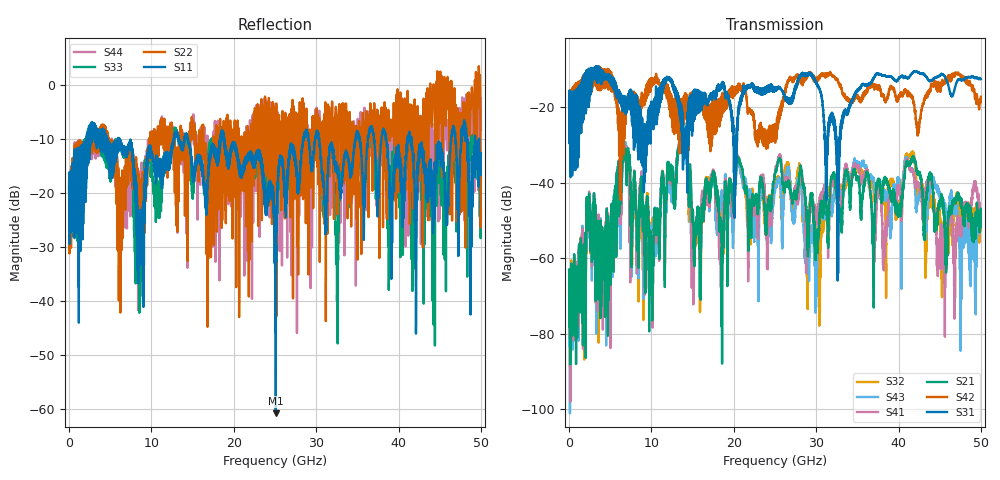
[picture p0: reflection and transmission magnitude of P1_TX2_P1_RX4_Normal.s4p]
!Keysight Technologies,N5225B,MY57041031,A.13.20.10
!Date: Friday, May 31, 2019 11:18:54
!Correction: S11(Full 4 Port(1,2,3,4))
!S12(Full 4 Port(1,2,3,4))
!S13(Full 4 Port(1,2,3,4))
!S14(Full 4 Port(1,2,3,4))
!S21(Full 4 Port(1,2,3,4))
!S22(Full 4 Port(1,2,3,4))
!S23(Full 4 Port(1,2,3,4))
!S24(Full 4 Port(1,2,3,4))
!S31(Full 4 Port(1,2,3,4))
!S32(Full 4 Port(1,2,3,4))
!S33(Full 4 Port(1,2,3,4))
!S34(Full 4 Port(1,2,3,4))
!S41(Full 4 Port(1,2,3,4))
!S42(Full 4 Port(1,2,3,4))
!S43(Full 4 Port(1,2,3,4))
!S44(Full 4 Port(1,2,3,4))
!S4P File: Measurements: <S11,S12,S13,S14>,
!<S21,S22,S23,S24>,
!<S31,S32,S33,S34>,
!<S41,S42,S43,S44>:
# Hz S  dB  R 50.0
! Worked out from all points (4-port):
!   5000 points, 10 MHz to 50 GHz, reference 50 ohm
!   strongest paths, dB at 10 MHz, 12.51 GHz, 25.01 GHz, 37.51 GHz, 50 GHz:
!     S31: -19.5, -13.0, -15.4, -11.1, -12.6
!     S42: -19.3, -19.5, -26.1, -14.9, -17.3
!     S21: -63.0, -38.6, -37.9, -39.2, -47.6
!     S41: -65.3, -39.8, -37.5, -42.3, -48.5
!     S43: -66.8, -44.0, -42.1, -42.7, -48.7
!     S32: -68.5, -42.4, -40.1, -39.7, -50.0
!   lowest |S11| = -60.7 dB at 25.1 GHz (marker M1), VSWR 1.00, Z = 49.9 - j0.0116 ohm
!   |S11| at or under -10 dB: 6.091 GHz to 12.71 GHz (6.616 GHz wide, 70.4 % of centre); 18.82 GHz to 28.43 GHz (9.605 GHz wide, 40.7 % of centre); 41.58 GHz to 46.39 GHz (4.81 GHz wide, 10.9 % of centre)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
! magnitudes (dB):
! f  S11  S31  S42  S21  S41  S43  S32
! 10 MHz  -19.9  -19.5  -19.3  -63.0  -65.3  -66.8  -68.5
! 6.74 GHz  -12.2  -19.2  -25.0  -32.0  -32.2  -31.3  -30.7
! 9.94 GHz  -12.7  -22.3  -13.8  -62.3  -58.4  -56.5  -58.9
! 13.65 GHz  -11.0  -19.9  -18.4  -29.8  -29.0  -28.4  -29.1
! 15.1 GHz  -16.2  -15.8  -17.8  -51.7  -62.6  -64.7  -52.3
! 25.1 GHz  -60.7  -15.1  -24.5  -36.6  -35.8  -40.7  -39.1
! 50 GHz  -12.6  -12.6  -17.3  -47.6  -48.5  -48.7  -50.0
